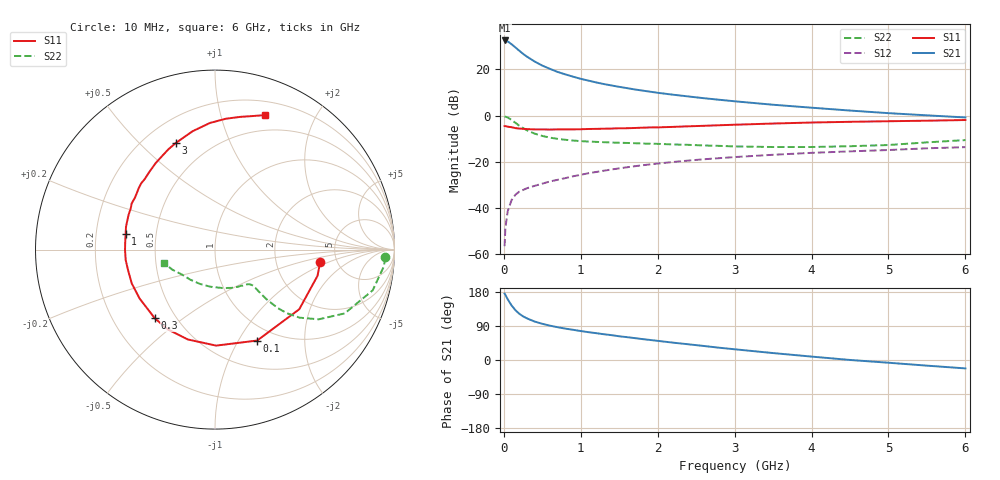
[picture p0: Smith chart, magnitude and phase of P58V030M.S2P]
! SIEMENS Small Signal Semiconductors
! BFP183
! Si NPN RF Bipolar Junction Transistor in SOT143
! VCE = 8 V  IC = 30 mA
! Common Emitter S-Parameters:  March  1996
# GHz  S  MA  R  50
!  f  S11  S21  S12  S22
! GHz  MAG  ANG  MAG  ANG  MAG  ANG  MAG  ANG
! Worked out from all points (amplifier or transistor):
!   36 points, 10 MHz to 6 GHz, reference 50 ohm
!   highest |S21| = 32.5 dB at 10 MHz (marker M1)
!   |S21| within 3 dB of that: start of sweep to 150.1 MHz
!   unconditionally stable (mu >= 1): 769.3 MHz to 5.73 GHz
!   at 250 MHz: K = 0.52, MSG = 29.4 dB, |S12| = -32.2 dB
!   at 1.4 GHz: K = 1.13, MAG = 16.0 dB, |S12| = -23.3 dB
!   at 6 GHz: K = 0.97, MSG = 6.4 dB, |S12| = -13.7 dB
!   S11 on the Smith chart (normalised r, x): 10 MHz: 3.70, -0.79; 100 MHz: 0.82, -1.20; 300 MHz: 0.38, -0.40; 1 GHz: 0.33, +0.08; 3 GHz: 0.33, +0.65; 6 GHz: 0.33, +1.39
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0.01  0.59 -6.8  41.95 175.2  0.0015 77.5  0.9502 -2.6
0.02  0.5896 -14.4  41.73 171.8  0.0037 78.7  0.9448 -5.8
0.05  0.5751 -35.3  40.03 160.3  0.0085 77.2  0.9074 -14.5
0.1  0.5585 -65.1  34.83 144.1  0.0148 63.6  0.8052 -26.2
0.15  0.535 -89.3  29.7 131.5  0.0194 57.1  0.6963 -33.9
0.2  0.5231 -106.9  25.24 122.2  0.0226 54.1  0.6053 -38.8
0.25  0.5164 -120.5  21.56 115.2  0.0246 51.1  0.5351 -41.5
0.3  0.5089 -131.2  18.78 109.9  0.0268 50.8  0.4803 -42.9
0.4  0.5008 -147.0  14.72 101.5  0.0302 50.9  0.4066 -43.9
0.5  0.5006 -157.9  11.99 95.5  0.0337 50.6  0.3617 -43.9
0.6  0.4977 -166.5  10.2 90.6  0.0376 51.8  0.3328 -43.7
0.7  0.501 -173.3  8.742 86.5  0.0408 53.1  0.3124 -43.5
0.8  0.5012 -179.7  7.745 82.8  0.0444 53.8  0.2991 -43.5
1  0.5052 170.2  6.213 76.4  0.0523 54.6  0.2797 -44.3
1.1  0.5117 165.7  5.679 73.4  0.0567 54.4  0.2736 -44.9
1.5  0.5308 151.0  4.169 62.6  0.0721 53.4  0.2581 -49.3
2.2  0.5681 129.7  2.819 45.8  0.0991 48.6  0.2372 -62.0
3  0.6326 110.3  2.032 28.3  0.1265 41.3  0.215 -82.0
3.5  0.6713 100.7  1.711 18.3  0.1418 36.8  0.2085 -96.9
4.5  0.7315 85.3  1.281 0.1  0.168 27.4  0.217 -129.6
5.5  0.7733 74.2  1.01 -14.9  0.1957 19.7  0.2628 -154.8
6  0.7996 69.6  0.908 -22.2  0.2072 15.2  0.2946 -165.6
